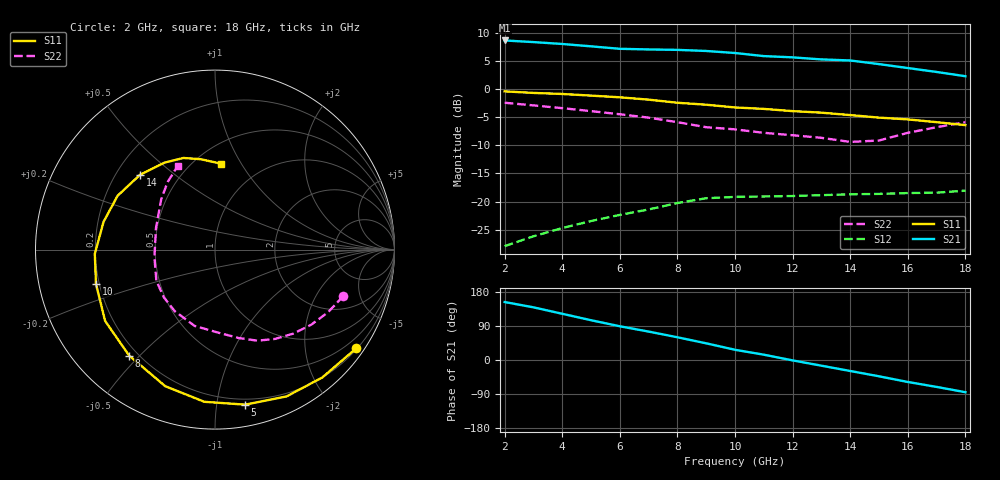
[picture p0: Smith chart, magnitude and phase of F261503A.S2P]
!ATF-26150
!S-PARAMETERS at Vds=3V  Id=10mA.  LAST UPDATED 07-22-92
# ghz s ma r 50
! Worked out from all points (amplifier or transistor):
!   17 points, 2 GHz to 18 GHz, reference 50 ohm
!   highest |S21| = 8.7 dB at 2 GHz (marker M1)
!   |S21| within 3 dB of that: start of sweep to 11.95 GHz
!   unconditionally stable (mu >= 1): 10.52 GHz to end of sweep
!   at 4 GHz: K = 0.33, MSG = 16.4 dB, |S12| = -24.7 dB
!   at 10 GHz: K = 0.96, MSG = 12.8 dB, |S12| = -19.2 dB
!   at 18 GHz: K = 1.58, MAG = 5.7 dB, |S12| = -18.1 dB
!   lowest NFmin = 1.30 dB at 6 GHz
!   S11 on the Smith chart (normalised r, x): 2 GHz: 0.22, -3.16; 5 GHz: 0.16, -1.20; 8 GHz: 0.17, -0.47; 10 GHz: 0.19, -0.14; 14 GHz: 0.30, +0.38; 18 GHz: 0.66, +0.82
2  0.96 -35.0  2.73 153.0  0.04 73.0  0.76 -20.0
3  0.93 -50.0  2.64 139.0  0.049 62.0  0.72 -29.0
4  0.91 -64.0  2.54 122.0  0.058 51.0  0.68 -38.0
5  0.88 -79.0  2.42 105.0  0.067 40.0  0.64 -47.0
6  0.85 -94.0  2.3 89.0  0.076 29.0  0.6 -56.0
7  0.81 -110.0  2.27 75.0  0.085 18.0  0.56 -65.0
8  0.76 -129.0  2.25 60.0  0.097 7.0  0.51 -75.0
9  0.73 -147.0  2.2 44.0  0.107 -3.0  0.46 -89.0
10  0.69 -164.0  2.11 27.0  0.11 -14.0  0.44 -105.0
11  0.67 -178.0  1.98 14.0  0.111 -20.0  0.41 -123.0
12  0.64 166.0  1.93 -1.0  0.112 -30.0  0.39 -137.0
13  0.62 151.0  1.85 -15.0  0.114 -32.0  0.37 -152.0
14  0.59 135.0  1.81 -29.0  0.116 -46.0  0.34 -173.0
15  0.56 120.0  1.68 -43.0  0.117 -54.0  0.35 160.0
16  0.54 109.0  1.55 -58.0  0.119 -67.0  0.41 137.0
17  0.51 99.0  1.43 -71.0  0.12 -72.0  0.46 125.0
18  0.48 86.0  1.31 -85.0  0.125 -77.0  0.51 114.0
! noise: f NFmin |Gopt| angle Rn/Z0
6  1.3  0.59  74  0.77
8  1.5  0.57  110  0.56
12  1.8  0.63  178  0.06
14  2  0.7  -134  0.73
